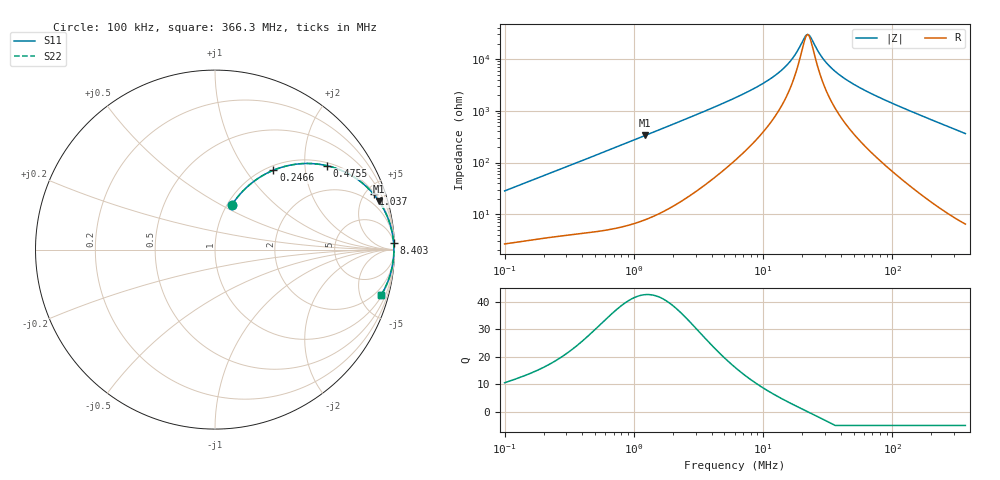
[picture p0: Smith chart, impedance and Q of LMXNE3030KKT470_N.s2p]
! LMXNE3030KKT470_N  S-PARAMETER MODEL  ( General Type )
! Model Generated by TAIYO YUDEN Corporation (http://www.ty-top.com)
! Version 1.0
! TAIYO YUDEN Control No. 191023NI43SB-FBB
! Copyright(c) 2019 TAIYO YUDEN CO.,LTD. All Rights Reserved.
! Product Description (link to TY-COMPAS)
! https://ds.yuden.co.jp/TYCOMPAS/or/detail?pn=LMXNE3030KKT470MN&u=M
! Products Name : Inductors
! Characteristics :
!  Inductance : 47 uH , SRF(min) : 17 MHz , DC Resistance(max) : 2.46 Ohm
!  Rated Current : Saturation :250 mA , Temp Rise : 285 mA
!  Case Size : 3.0 x 3.0 / 0.118 x 0.118 [mm/inch] , Thickness : 1 / 0.039 [mm/inch]
!  (Conditions: Temperature = 25 degC , DC Bias Current/Voltage = 0A / 0V)
! External Node Assignments :
!  1  o---GGG---o  2
! GND o---------o GND
! Frequency Range : 0.1MHz  -  366.261039MHz  [ 402 STEP ]
# MHz S RI R 50
! Freq[MHz].  S11 Real  S11 Imag  S21 Real  S21 Imag  S12 Real  S12 Imag  S22 Real  S22 Imag
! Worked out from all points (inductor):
!   401 points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, 100 kHz to 366.3 MHz, reference 50 ohm
!   read as one part in series: L = 44.6 uH near 104.2 kHz
!   highest Q = 42.6 at 1.222 MHz (marker M1), where L = 43.5 uH
!   self-resonance near 22.04 MHz
!   S11 on the Smith chart (normalised r, x): 100 kHz: 1.05, +0.56; 246.6 kHz: 1.07, +1.36; 475.5 kHz: 1.09, +2.60; 1.037 MHz: 1.14, +5.66; 8.403 MHz: 6, +53; 366.3 MHz: 1.13, -7.27
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0.1  0.0941 0.2483  0.9059 -0.2483  0.9059 -0.2483  0.0941 0.2483
0.160294  0.1836 0.3533  0.8164 -0.3533  0.8164 -0.3533  0.1836 0.3533
0.246614  0.3259 0.4424  0.6741 -0.4424  0.6741 -0.4424  0.3259 0.4424
0.395307  0.5386 0.4793  0.4614 -0.4793  0.4614 -0.4793  0.5386 0.4793
0.475467  0.6245 0.4673  0.3755 -0.4673  0.3755 -0.4673  0.6245 0.4673
0.702102  0.7798 0.4009  0.2202 -0.4009  0.2202 -0.4009  0.7798 0.4009
1.036765  0.8833 0.3094  0.1167 -0.3094  0.1167 -0.3094  0.8833 0.3094
1.221676  0.9123 0.2714  0.0877 -0.2714  0.0877 -0.2714  0.9123 0.2714
1.562679  0.9434 0.2194  0.0566 -0.2194  0.0566 -0.2194  0.9434 0.2194
6.177387  0.9936 0.0543  0.00642 -0.0543  0.00642 -0.0543  0.9936 0.0543
8.403244  0.9952 0.0371  0.00477 -0.0371  0.00477 -0.0371  0.9952 0.0371
11.66806  0.9961 0.0225  0.00386 -0.0225  0.00386 -0.0225  0.9961 0.0225
14.92493  0.9965 0.0133  0.00352 -0.0133  0.00352 -0.0133  0.9965 0.0133
17.58685  0.9966 0.00759  0.00339 -0.00759  0.00339 -0.00759  0.9966 0.00759
21.59151  0.9967 0.000738  0.00333 -0.000738  0.00333 -0.000738  0.9967 0.000738
22.49582  0.9967 -0.000619  0.00333 0.000619  0.00333 0.000619  0.9967 -0.000619
23.92381  0.9967 -0.00266  0.00333 0.00266  0.00333 0.00266  0.9967 -0.00266
29.37143  0.9966 -0.00957  0.00342 0.00957  0.00342 0.00957  0.9966 -0.00957
37.56979  0.9963 -0.0184  0.00367 0.0184  0.00367 0.0184  0.9963 -0.0184
54.35123  0.9955 -0.0339  0.0045 0.0339  0.0045 0.0339  0.9955 -0.0339
94.57258  0.9921 -0.0666  0.00789 0.0666  0.00789 0.0666  0.9921 -0.0666
366.261  0.9258 -0.2534  0.0742 0.2534  0.0742 0.2534  0.9258 -0.2534
